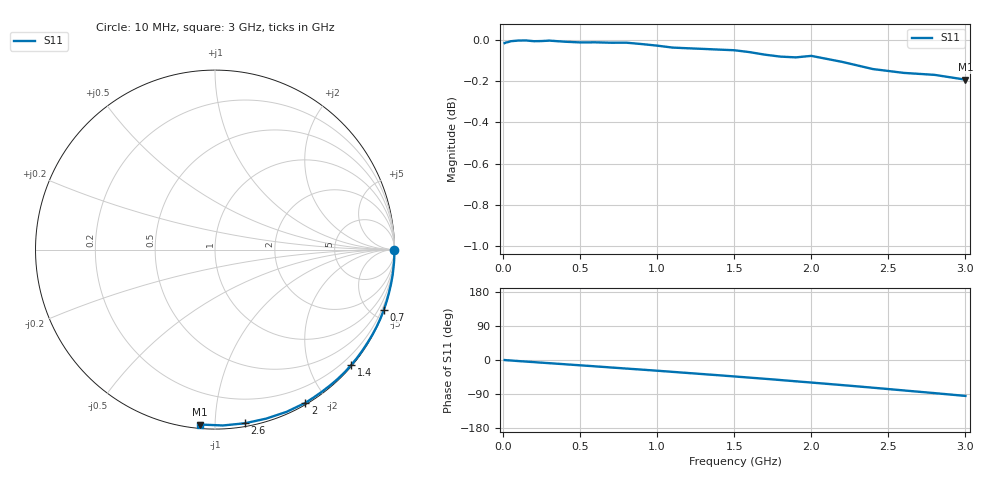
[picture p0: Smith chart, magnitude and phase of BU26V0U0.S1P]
! SIEMENS Small Signal Semiconductors
! BB833
! Si Tuning Diode in SOD323
! VR = 26 V
! S-Parameters:  April  1996
# GHz  S  MA  R  50
!  f  S11
! GHz  MAG  ANG
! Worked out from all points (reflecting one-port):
!   31 points, 10 MHz to 3 GHz, reference 50 ohm
!   lowest |S11| = -0.2 dB at 3 GHz (marker M1), VSWR 90.62, Z = 1.02 - j46 ohm
!   phase of S11 starts at -0 deg and turns -95 deg over the sweep
!   S11 on the Smith chart (normalised r, x): 10 MHz: open; 700 MHz: 0.02, -5.76; 1.4 GHz: 0.02, -2.73; 2 GHz: 0.02, -1.75; 2.6 GHz: 0.02, -1.19; 3 GHz: 0.02, -0.92
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0.01  0.9984 -0.1
0.02  0.9988 -0.5
0.03  0.9989 -0.8
0.05  0.9994 -1.3
0.1  0.9998 -2.8
0.15  0.9999 -4.2
0.3  0.9998 -8.4
0.4  0.9992 -11.2
0.5  0.9988 -14.0
0.6  0.9988 -16.8
0.7  0.9986 -19.7
0.8  0.9986 -22.6
0.9  0.9978 -25.4
1  0.997 -28.3
1.2  0.9955 -34.3
1.3  0.9951 -37.3
1.4  0.9948 -40.3
1.5  0.9944 -43.4
1.6  0.9933 -46.5
1.7  0.9919 -49.6
1.8  0.9909 -52.9
1.9  0.9904 -56.2
2  0.9913 -59.5
2.2  0.9879 -66.2
2.4  0.984 -73.1
2.6  0.9819 -80.3
2.8  0.9808 -87.4
3  0.9782 -94.8
